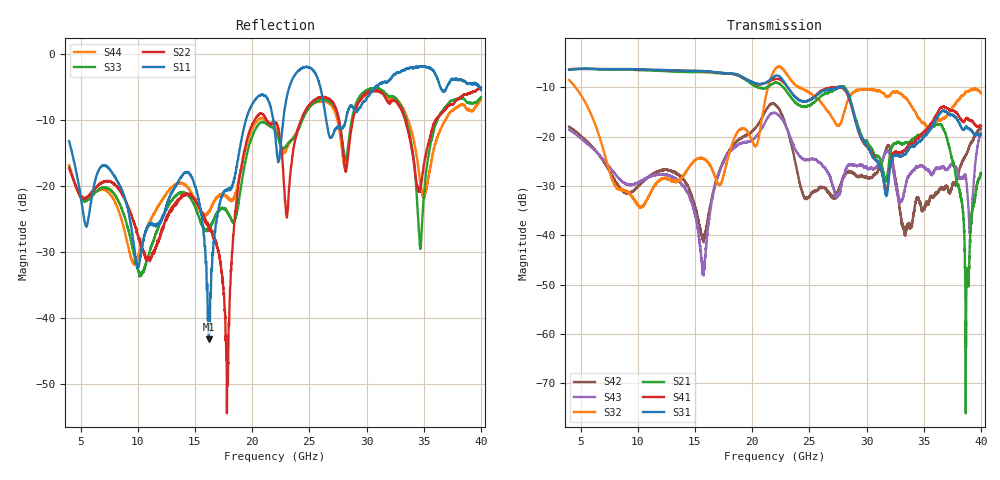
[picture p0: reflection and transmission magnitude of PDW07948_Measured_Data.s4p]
!The following data was pulled from an Agilent PNA
!This sNp file was generated from the data in the RF Test software
!NOTE:  Smoothing/Math/Corrections applied on any given trace ARE included in the data saved here
# MHz S dB R 50
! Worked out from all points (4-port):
!   6401 points, 4 GHz to 40 GHz, reference 50 ohm
!   strongest paths, dB at 4 GHz, 13 GHz, 22 GHz, 31 GHz, 40 GHz:
!     S31: -6.5, -6.6, -7.7, -25.3, -19.6
!     S41: -6.4, -6.6, -8.3, -25.2, -17.8
!     S21: -6.4, -6.8, -9.1, -24.0, -27.3
!     S32: -8.5, -29.0, -6.3, -10.7, -11.3
!     S43: -18.6, -28.1, -15.2, -25.7, -19.2
!     S42: -18.0, -27.0, -13.5, -26.9, -18.5
!   lowest |S11| = -43.2 dB at 16.22 GHz (marker M1), VSWR 1.01, Z = 49.6 - j0.564 ohm
!   |S11| at or under -10 dB: start of sweep to 19.46 GHz; 21.85 GHz to 22.72 GHz (872.8 MHz wide, 3.92 % of centre); 26.48 GHz to 28.2 GHz (1.719 GHz wide, 6.29 % of centre)
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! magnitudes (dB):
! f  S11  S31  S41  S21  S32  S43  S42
! 4 GHz  -13.3  -6.5  -6.4  -6.4  -8.5  -18.6  -18.0
! 16.22 GHz  -43.2  -6.8  -6.9  -7.0  -25.5  -37.2  -35.5
! 17.84 GHz  -20.5  -7.2  -7.2  -7.3  -24.8  -23.8  -23.5
! 20.53 GHz  -6.4  -9.3  -9.4  -10.0  -20.8  -19.5  -17.6
! 36.54 GHz  -5.3  -15.0  -14.1  -17.6  -16.5  -26.1  -30.4
! 38.8 GHz  -4.5  -18.1  -16.3  -46.9  -10.9  -30.6  -23.2
! 40 GHz  -5.5  -19.6  -17.8  -27.3  -11.3  -19.2  -18.5
